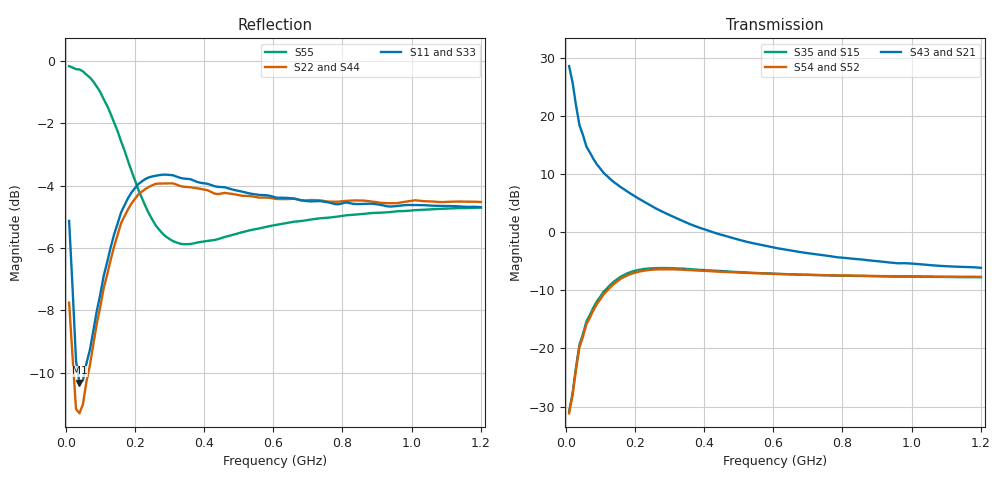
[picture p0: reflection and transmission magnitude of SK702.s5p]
!  POLYFET RF DEVICES
!  S PARAMETERS FOR
!  SK702 (EACH SIDE)
!  VDS=28, IDQ=400MA
! S1A2Die, Vds=28Vdc, Idq=400ma, Vgsth=2.63Vdc
! Date: Thu Jul 23 11:52:17 1998
!AWR Design Environment (2053) Wed Feb 04 15:36:44 2004
!freq-unit  param-type  data-format  keyword  impedance-ohms
# MHz  S  MA  R  50
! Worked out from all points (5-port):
!   120 points, 10 MHz to 1.2 GHz, reference 50 ohm
!   strongest paths, dB at 10 MHz, 310 MHz, 610 MHz, 910 MHz, 1.2 GHz:
!     S43: 28.5, 2.7, -2.7, -5.0, -6.1
!     S21: 28.5, 2.7, -2.7, -5.0, -6.1
!     S54: -31.2, -6.4, -7.2, -7.5, -7.7
!     S52: -31.2, -6.4, -7.2, -7.5, -7.7
!     S35: -30.8, -6.2, -7.2, -7.6, -7.8
!     S15: -30.8, -6.2, -7.2, -7.6, -7.8
!   lowest |S11| = -10.3 dB at 40 MHz (marker M1), VSWR 1.88, Z = 49.3 - j31.8 ohm
!   |S11| at or under -10 dB: 35.47 MHz to 54.49 MHz (19.02 MHz wide, 42.3 % of centre)
